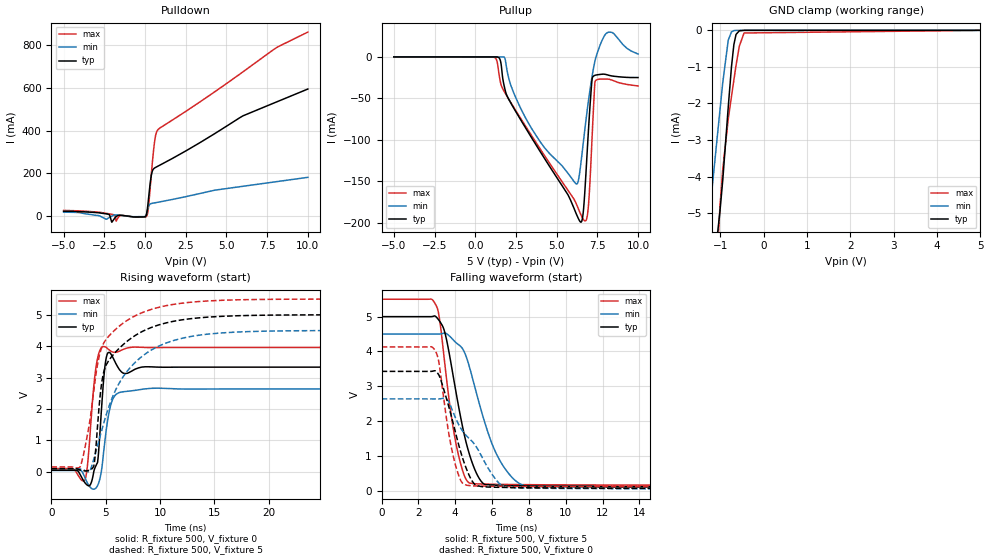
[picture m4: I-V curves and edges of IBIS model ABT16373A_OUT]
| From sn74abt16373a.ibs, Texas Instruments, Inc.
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[Model]   ABT16373A_OUT
Model_type  3-state
Enable   Active-Low
Vref =   0
Rref =   500
Cref =   50p
Vmeas =   1.5
| variable   typ   min   max
C_comp   5.59pF   4.99pF   6.42pF
| C_pullup   6.48pF   2.62pF   8.96pF
| C_pulldown   20.34pF   3.16pF   55.47pF
| C_tri-state   5.59pF   4.99pF   6.42pF
[Temperature Range]   40   -40   100
| Ambient temperature   25   -40   85
[Voltage range]   5   4.5   5.5
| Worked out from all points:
|   slope of the pulldown table from 0 to 0.75 V, typ, clamps not added: 3.19 ohm
|   GND clamp passes 1 mA (typ) near -0.75 V on its own axis
|   rising waveform, R_fixture 500, V_fixture 0: 20-80 % time 389ps typ, 671ps min, 560ps max; typ from 0.049 V to 3.33 V
|   falling waveform, R_fixture 500, V_fixture 5: 20-80 % time 1.1ns typ, 1.58ns min, 824ps max; typ from 5 V to 0.097 V
|   rising waveform, R_fixture 500, V_fixture 5: 20-80 % time 2.34ns typ, 3.78ns min, 2.25ns max; typ from 0.094 V to 5 V
|   falling waveform, R_fixture 500, V_fixture 0: 20-80 % time 1.07ns typ, 1.89ns min, 719ps max; typ from 3.43 V to 0.051 V
[GND Clamp]
| ABT16373A_OUT
|   Voltage   I(typ)   I(min)   I(max)
-5V       -407.1mA   -371.1mA   -431.8mA
-1.285V   -7.755mA   -5.399mA   -16.3mA
-1.065V   -5.534mA   -2.818mA   -5.984mA
-1.01V    -4.938mA   -2.167mA   -4.801mA
-945mV    -4.074mA   -1.414mA   -3.784mA
-820mV    -2.099mA   -269.1uA   -2.433mA
-745mV    -991.6uA   -40.48uA   -1.809mA
-690mV    -390.6uA   -8.4uA     -1.361mA
-640mV    -111.8uA   -1.718uA   -958.8uA
-565mV    -14.53uA   -178.5nA   -436.3uA
-455mV    -478.7nA   -8.271nA   -72.81uA
5V        148pA      155.7pA    3.546nA
[Pulldown]
| ABT16373A_OUT
|   Voltage   I(typ)   I(min)   I(max)
-5V       22.55mA    18.36mA    26.32mA
-2.285V   8.949mA    -11.18mA   11.43mA
-2.04V    -28.8mA    -220uA     8.321mA
-1.77V    -2.584mA   5.546mA    -23.31mA
-1.465V   3.422mA    3.146mA    3.124mA
75mV      4.31mA     5.695mA    -2.48mA
200mV     71.07mA    41.73mA    34.45mA
435mV     207.1mA    59.54mA    237.3mA
625mV     226.8mA    62.28mA    367.2mA
810mV     234.4mA    64.89mA    405.9mA
6.03V     470.1mA    139.6mA    676.5mA
10V       595.2mA    181.4mA    862mA
[Pullup]
| ABT16373A_OUT
|   Voltage   I(typ)   I(min)   I(max)
-5V       -13.59pA   -8.413pA   24.5pA
1.455V    -937.1uA   -30.81pA   -19.94mA
1.955V    -46.95mA   -16.51mA   -47.47mA
4.245V    -121.9mA   -109.1mA   -118.4mA
6.21V     -189.2mA   -153.1mA   -177mA
6.485V    -199mA     -129mA     -189.8mA
6.66V     -181.9mA   -99.56mA   -196.2mA
6.9V      -106.4mA   -60.9mA    -189.2mA
7.2V      -24.8mA    -20.91mA   -87.48mA
7.405V    -21.89mA   -1.038mA   -28.27mA
8.23V     -22.26mA   29.88mA    -26.91mA
10V       -24.86mA   3.458mA    -34.96mA
[Ramp]
| ABT16373A_OUT
| variable   typ   min   max
dV/dt_r   2.55/5.48E-10   1.93/7.83E-10   2.57/6.23E-10
dV/dt_f   2.95/1.11E-09   2.67/1.60E-09   3.21/8.28E-10
R_load = 500
[Rising Waveform]
| ABT16373A_OUT
R_fixture =   500
C_fixture =   0
L_fixture =   0
V_fixture =   0
V_fixture_min = 0
V_fixture_max = 0
|   Time   V(typ)   V(min)   V(max)
0s        49.18mV    41.04mV    103mV
3.09ns    -350.4mV   -189.2mV   -261.4mV
3.58ns    -413.8mV   -493.7mV   1.308V
3.94ns    56.24mV    -551.8mV   2.857V
4.245ns   293.3mV    -442.3mV   3.607V
4.74ns    2.632V     403.8mV    3.99V
5.22ns    3.793V     1.729V     3.908V
5.725ns   3.593V     2.365V     3.807V
6.625ns   3.139V     2.55V      3.898V
50ns      3.333V     2.637V     3.958V
[Falling Waveform]
| ABT16373A_OUT
R_fixture =   500
C_fixture =   0
L_fixture =   0
V_fixture =   5
V_fixture_min = 4.5
V_fixture_max = 5.5
|   Time   V(typ)   V(min)   V(max)
0s        5V         4.5V       5.5V
2.975ns   4.987V     4.498V     5.307V
3.445ns   4.523V     4.528V     3.59V
4.015ns   2.908V     4.265V     1.422V
4.465ns   1.669V     4.014V     473mV
4.81ns    974.5mV    3.478V     211.5mV
5.465ns   232.7mV    2.202V     189.1mV
6.235ns   154.6mV    1.055V     180.8mV
7.91ns    135mV      124mV      170.8mV
50ns      96.58mV    87.76mV    153.1mV
[Rising Waveform]
| ABT16373A_OUT
R_fixture =   500
C_fixture =   0
L_fixture =   0
V_fixture =   5
V_fixture_min = 4.5
V_fixture_max = 5.5
|   Time   V(typ)   V(min)   V(max)
0s        94.44mV    87.28mV    153mV
2.635ns   59.33mV    88.43mV    154.3mV
3.805ns   124.1mV    291.9mV    2.329V
4.01ns    452.5mV    535.3mV    2.87V
4.575ns   2.689V     1.248V     3.899V
5ns       3.372V     1.761V     4.194V
6.615ns   4.053V     3.033V     4.736V
9.17ns    4.592V     3.872V     5.168V
17.18ns   4.969V     4.452V     5.476V
50ns      5V         4.5V       5.5V
[Falling Waveform]
| ABT16373A_OUT
R_fixture =   500
C_fixture =   0
L_fixture =   0
V_fixture =   0
V_fixture_min = 0
V_fixture_max = 0
|   Time   V(typ)   V(min)   V(max)
0s        3.427V     2.636V     4.129V
2.9ns     3.444V     2.636V     4.031V
3.105ns   3.327V     2.635V     3.704V
3.925ns   1.856V     2.201V     919.2mV
4.29ns    1.124V     1.801V     298.2mV
4.66ns    555.9mV    1.547V     150.1mV
5.175ns   141.2mV    1.233V     133.7mV
6.265ns   95.98mV    279.9mV    124.4mV
6.975ns   89.58mV    81.21mV    120.5mV
50ns      51.04mV    41.72mV    103mV
